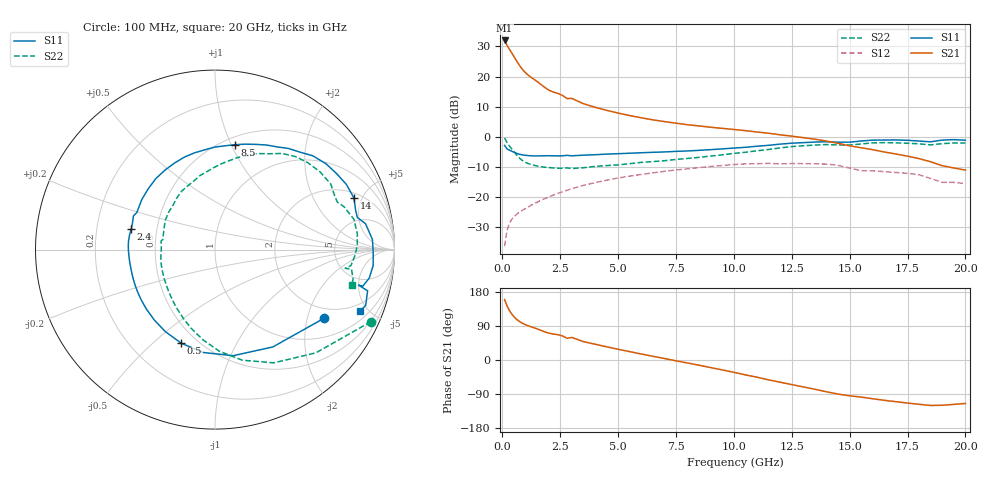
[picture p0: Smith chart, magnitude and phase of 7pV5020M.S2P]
! Infineon Technologies  Discrete & RF Semiconductors
! bfp620
! VCE = 0.50 V,  IC =  20 mA
! Common Emitter S-Parameters:  Sep 2002
# GHz  S  MA  R  50
!  f  S11  S21  S12  S22
! GHz  MAG  ANG  MAG  ANG  MAG  ANG  MAG  ANG
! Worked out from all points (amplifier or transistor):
!   59 points, 100 MHz to 20 GHz, reference 50 ohm
!   highest |S21| = 32.0 dB at 100 MHz (marker M1)
!   |S21| within 3 dB of that: start of sweep to 314.3 MHz
!   unconditionally stable (mu >= 1): 3.273 GHz to 10.06 GHz; 17.14 GHz to end of sweep
!   at 1 GHz: K = 0.71, MSG = 22.6 dB, |S12| = -23.8 dB
!   at 5.5 GHz: K = 1.05, MAG = 8.7 dB, |S12| = -13.1 dB
!   at 20 GHz: K = 1.64, MAG = -2.4 dB, |S12| = -15.6 dB
!   S11 on the Smith chart (normalised r, x): 100 MHz: 1.61, -2.55; 500 MHz: 0.41, -0.62; 2.4 GHz: 0.36, +0.11; 8.5 GHz: 0.57, +1.03; 14 GHz: 2.37, +4.30; 20 GHz: 1.49, -4.44
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0.1  0.7179 -32.2  39.84 159.3  0.0152 74.2  0.9572 -24.8
0.2  0.6309 -59.3  33.35 143.7  0.0272 62.1  0.804 -45.7
0.3  0.5996 -80.3  28.78 131.4  0.0358 56.6  0.7106 -62.6
0.4  0.577 -96.5  24.98 121.9  0.042 52.9  0.6349 -76.1
0.5  0.5545 -109.8  21.62 114.4  0.0468 50.3  0.567 -87.5
0.6  0.5341 -121.2  18.7 108.4  0.0508 48.5  0.5076 -97.5
0.7  0.5178 -130.9  16.26 103.5  0.0543 47.4  0.4592 -106.6
0.8  0.5059 -139.1  14.29 99.4  0.0576 46.7  0.422 -114.7
1  0.4916 -151.2  11.61 93.1  0.0642 46.4  0.375 -127.6
1.8  0.4825 -179.9  6.761 75.1  0.0924 45.5  0.313 -161.6
2.4  0.4806 166.3  5.245 66.8  0.1146 42.9  0.2999 -177.7
2.8  0.4916 157.5  4.304 57.2  0.1295 40.1  0.3041 170.7
3  0.4822 154.6  4.342 59.6  0.137 38.8  0.2961 169.1
3.5  0.4943 145.5  3.546 48.6  0.1553 34.7  0.3056 158.7
5  0.523 122.3  2.475 28.3  0.2064 21.2  0.3405 133.4
7  0.5595 95.5  1.787 4.0  0.2663 2.2  0.3995 107.2
8.5  0.5948 79.3  1.512 -13.8  0.3072 -13.0  0.4549 91.4
10.5  0.6684 58.9  1.262 -39.3  0.3542 -36.6  0.5527 71.1
13.5  0.8172 26.4  0.91 -77.2  0.3549 -72.1  0.7281 36.5
14  0.8258 20.4  0.849 -83.8  0.3518 -79.0  0.7412 29.5
17  0.8856 -5.8  0.517 -110.0  0.2548 -103.3  0.793 1.5
20  0.8776 -23.0  0.28 -114.7  0.1669 -114.8  0.7865 -14.5
